ORGANIZATION_BLOCK "Restart"
TITLE = "Complete Restart"
AUTHOR : MassimoZ
FAMILY : NovaSrl
VERSION : 0.1


VAR_TEMP
  OB100_EV_CLASS : BYTE ;	//16#13, Event class 1, Entering event state, Event logged in diagnostic buffer
  OB100_STRTUP : BYTE ;	//16#81/82/83/84 Method of startup
  OB100_PRIORITY : BYTE ;	//27 (Priority of 1 is lowest)
  OB100_OB_NUMBR : BYTE ;	//100 (Organization block 100, OB100)
  OB100_RESERVED_1 : BYTE ;	//Reserved for system
  OB100_RESERVED_2 : BYTE ;	//Reserved for system
  OB100_STOP : WORD ;	//Event that caused CPU to stop (16#4xxx)
  OB100_STRT_INFO : DWORD ;	//Information on how system started
  OB100_DATE_TIME : DATE_AND_TIME ;	//Date and time OB100 started
END_VAR
BEGIN
NETWORK
TITLE =Caricamento Output sulla DB100

      U(    ;
      U(    ;
      L     "Gest Stato Output".StatoOutputByte16_17;
      T     AW    16;
      SET   ;
      SAVE  ;
      CLR   ;
      U     BIE;
      )     ;
      SPBNB _001;
      L     "Gest Stato Output".StatoOutputByte18_19;
      T     AW    18;
      SET   ;
      SAVE  ;
      CLR   ;
_001: U     BIE;
      )     ;
      SPBNB _002;
      L     "Gest Stato Output".StatoOutputByte20_21;
      T     AW    20;
_002: NOP   0;
NETWORK
TITLE =Caricamento Output sulla DB100

      L     "Gest Stato Output".StatoOutputByte22_23;
      T     AW    22;
      NOP   0;
NETWORK
TITLE =Caricamento Quota Base Asse X

      L     L#0;
      T     "Scambio dati OP".QuotaBaseAsseX;
      NOP   0;
NETWORK
TITLE =Caricamento Quota Base Asse Y

      L     L#0;
      T     "Scambio dati OP".QuotaBaseAsseY;
      NOP   0;
END_ORGANIZATION_BLOCK

